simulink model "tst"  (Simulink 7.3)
settings: Solver=ode45  StartTime=0.0  StopTime=10.0  RelTol=1e-3
undefined symbols (not defined in the file or in its folder): Acl, Bcl, Ccl, Dcl

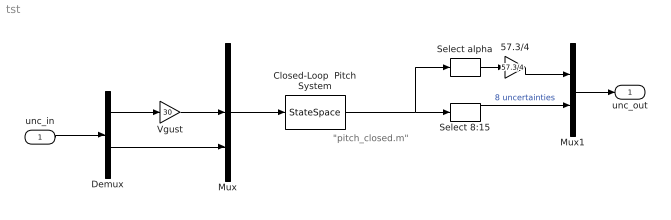
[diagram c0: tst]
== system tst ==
  note: "pitch_closed.m"
  unc_in : Inport
  57.3/4 : Gain  Gain=57.3/4  ParameterDataType=fixdt(1, 16)  ParameterScaling=2^0  OutDataType=fixdt(1, 16)  OutScaling=2^0
  Closed-Loop  Pitch System : StateSpace  A=Acl  B=Bcl  C=Ccl  D=Dcl
  Demux : Demux  Outputs=[1,8]
  Mux : Mux  Inputs=[1, 1, 8]
  Mux1 : Mux  Inputs="[1,  8]"
  Select 8:15 : Selector  InputPortWidth=15  IndexOptions=Index vector (dialog)  Indices=[8:15]  OutputSizes=1
  Select alpha : Selector  InputPortWidth=15  IndexOptions=Index vector (dialog)  Indices=[5]  OutputSizes=1
  Vgust : Gain  Gain=30  ParameterDataType=fixdt(1, 16)  ParameterScaling=2^0  OutDataType=fixdt(1, 16)  OutScaling=2^0
  unc_out : Outport
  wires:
  Closed-Loop  Pitch System/1 -> Select alpha/1, Select 8:15/1
  Select 8:15/1 -> Mux1/2  "8 uncertainties"
  Select alpha/1 -> 57.3/4/1
  Mux1/1 -> unc_out/1
  57.3/4/1 -> Mux1/1
  Mux/1 -> Closed-Loop  Pitch System/1
  unc_in/1 -> Demux/1
  Demux/2 -> Mux/3
  Demux/1 -> Vgust/1
  Vgust/1 -> Mux/2
